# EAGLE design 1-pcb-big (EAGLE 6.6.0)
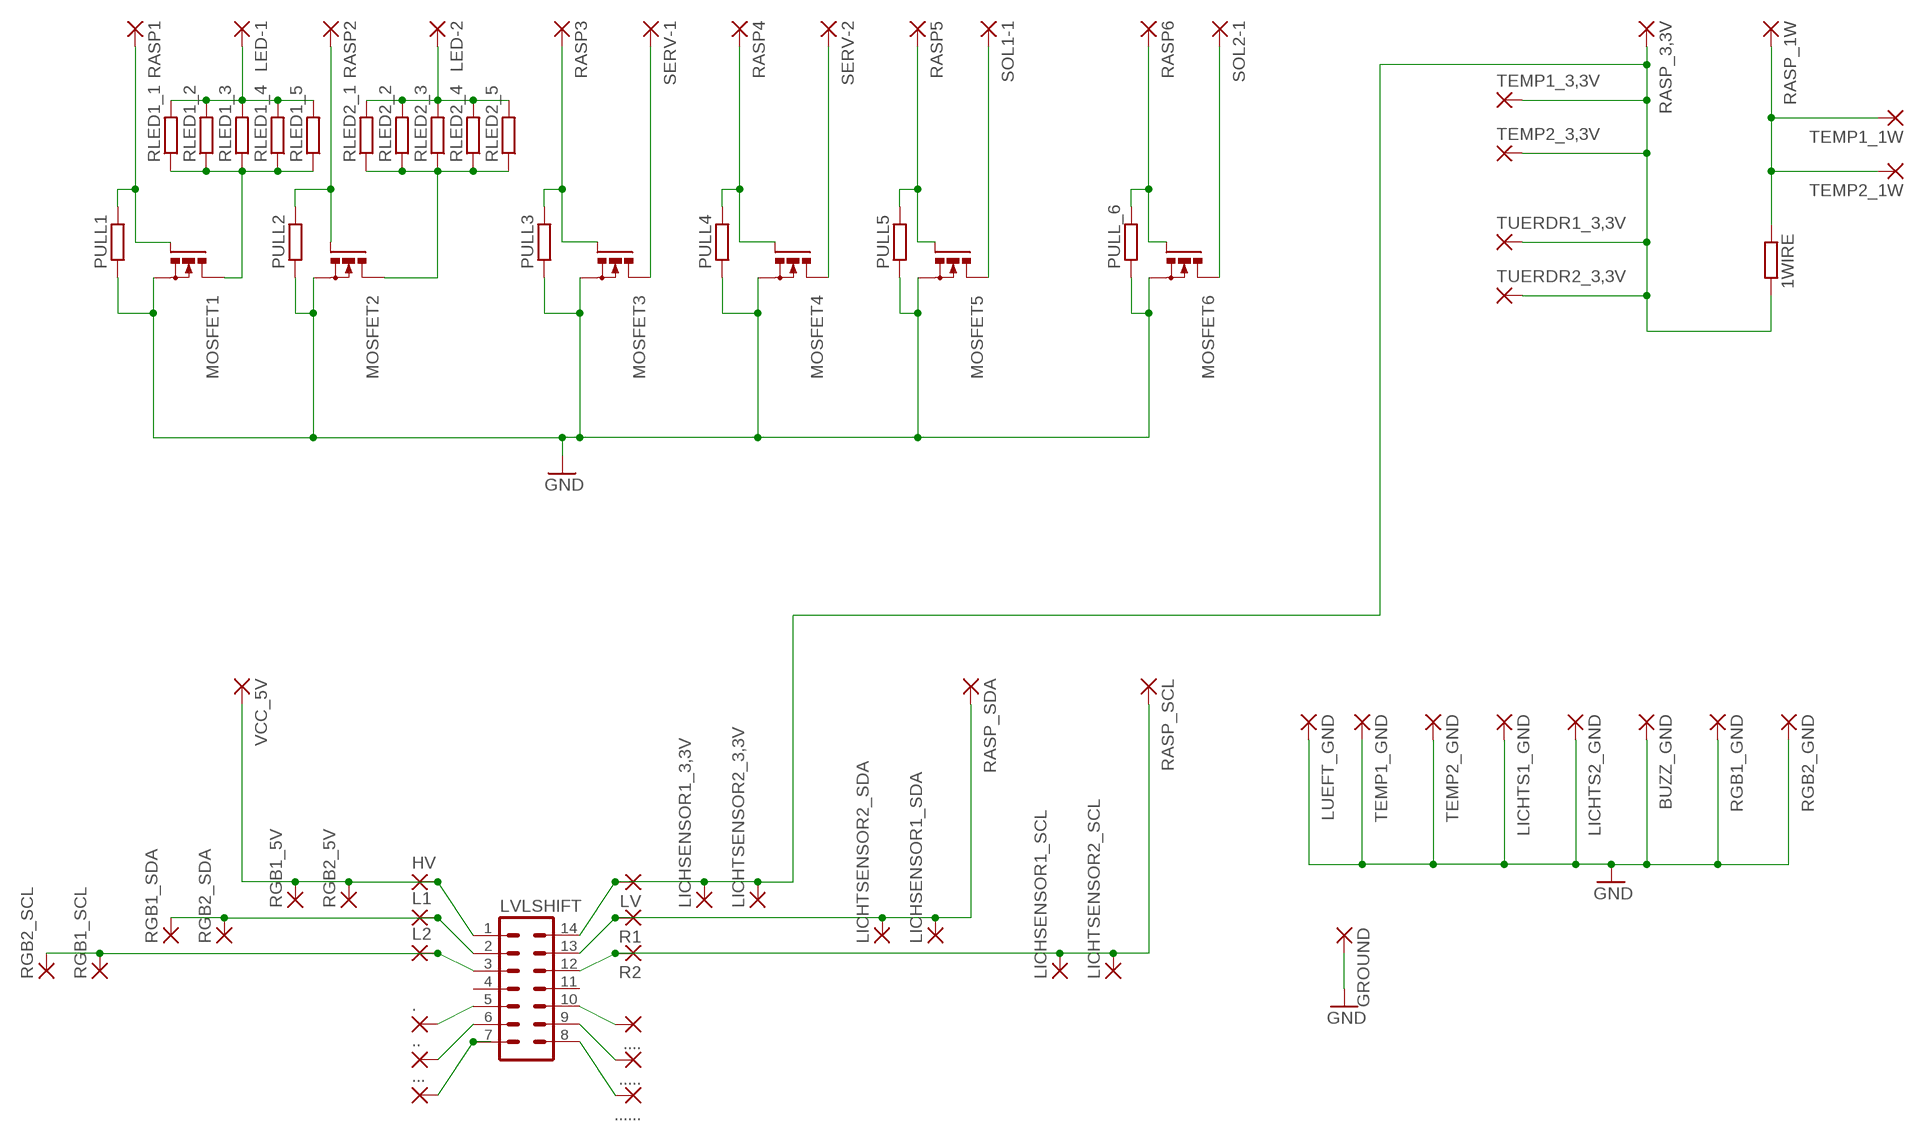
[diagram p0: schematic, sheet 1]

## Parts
1WIRE  R-EU_0207/15  [0207/15]
.  2,15/1,0  [2,15/1,0]
..  2,15/1,0  [2,15/1,0]
...  2,15/1,0  [2,15/1,0]
....  2,15/1,0  [2,15/1,0]
.....  2,15/1,0  [2,15/1,0]
......  2,15/1,0  [2,15/1,0]
BUZZ_GND  2,15/1,0  [2,15/1,0]
GROUND  2,15/1,0  [2,15/1,0]
HV  2,15/1,0  [2,15/1,0]
L1  2,15/1,0  [2,15/1,0]
L2  2,15/1,0  [2,15/1,0]
LED-1  2,15/1,0  [2,15/1,0]
LED-2  2,15/1,0  [2,15/1,0]
LICHSENSOR1_3,3V  2,15/1,0  [2,15/1,0]
LICHSENSOR1_SCL  2,15/1,0  [2,15/1,0]
LICHSENSOR1_SDA  2,15/1,0  [2,15/1,0]
LICHTS1_GND  2,15/1,0  [2,15/1,0]
LICHTS2_GND  2,15/1,0  [2,15/1,0]
LICHTSENSOR2_3,3V  2,15/1,0  [2,15/1,0]
LICHTSENSOR2_SCL  2,15/1,0  [2,15/1,0]
LICHTSENSOR2_SDA  2,15/1,0  [2,15/1,0]
LUEFT_GND  2,15/1,0  [2,15/1,0]
LV  2,15/1,0  [2,15/1,0]
LVLSHIFT  IC14P  [IC14P]
MOSFET1  BUZ11BV  [TO220BV]
MOSFET2  BUZ11BV  [TO220BV]
MOSFET3  BUZ11BV  [TO220BV]
MOSFET4  BUZ11BV  [TO220BV]
MOSFET5  BUZ11BV  [TO220BV]
MOSFET6  BUZ11BV  [TO220BV]
PULL1  R-EU_0207/10  [0207/10]
PULL2  R-EU_0207/10  [0207/10]
PULL3  R-EU_0207/10  [0207/10]
PULL4  R-EU_0207/10  [0207/10]
PULL5  R-EU_0207/10  [0207/10]
PULL_6  R-EU_0207/10  [0207/10]
R1  2,15/1,0  [2,15/1,0]
R2  2,15/1,0  [2,15/1,0]
RASP1  2,15/1,0  [2,15/1,0]
RASP2  2,15/1,0  [2,15/1,0]
RASP3  2,15/1,0  [2,15/1,0]
RASP4  2,15/1,0  [2,15/1,0]
RASP5  2,15/1,0  [2,15/1,0]
RASP6  2,15/1,0  [2,15/1,0]
RASP_1W  2,15/1,0  [2,15/1,0]
RASP_3,3V  2,15/1,0  [2,15/1,0]
RASP_SCL  2,15/1,0  [2,15/1,0]
RASP_SDA  2,15/1,0  [2,15/1,0]
RGB1_5V  2,15/1,0  [2,15/1,0]
RGB1_GND  2,15/1,0  [2,15/1,0]
RGB1_SCL  2,15/1,0  [2,15/1,0]
RGB1_SDA  2,15/1,0  [2,15/1,0]
RGB2_5V  2,15/1,0  [2,15/1,0]
RGB2_GND  2,15/1,0  [2,15/1,0]
RGB2_SCL  2,15/1,0  [2,15/1,0]
RGB2_SDA  2,15/1,0  [2,15/1,0]
RLED1_1  R-EU_0207/15  [0207/15]
RLED1_2  R-EU_0207/15  [0207/15]
RLED1_3  R-EU_0207/15  [0207/15]
RLED1_4  R-EU_0207/15  [0207/15]
RLED1_5  R-EU_0207/15  [0207/15]
RLED2_1  R-EU_0207/15  [0207/15]
RLED2_2  R-EU_0207/15  [0207/15]
RLED2_3  R-EU_0207/15  [0207/15]
RLED2_4  R-EU_0207/15  [0207/15]
RLED2_5  R-EU_0207/15  [0207/15]
SERV-1  2,15/1,0  [2,15/1,0]
SERV-2  2,15/1,0  [2,15/1,0]
SOL1-1  2,15/1,0  [2,15/1,0]
SOL2-1  2,15/1,0  [2,15/1,0]
TEMP1_1W  2,15/1,0  [2,15/1,0]
TEMP1_3,3V  2,15/1,0  [2,15/1,0]
TEMP1_GND  2,15/1,0  [2,15/1,0]
TEMP2_1W  2,15/1,0  [2,15/1,0]
TEMP2_3,3V  2,15/1,0  [2,15/1,0]
TEMP2_GND  2,15/1,0  [2,15/1,0]
TUERDR1_3,3V  2,15/1,0  [2,15/1,0]
TUERDR2_3,3V  2,15/1,0  [2,15/1,0]
VCC_5V  2,15/1,0  [2,15/1,0]

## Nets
GND: BUZZ_GND.1(P) GROUND.1(P) LICHTS1_GND.1(P) LICHTS2_GND.1(P) LUEFT_GND.1(P) MOSFET1.S MOSFET2.S MOSFET3.S MOSFET4.S MOSFET5.S MOSFET6.S PULL1.1 PULL2.1 PULL3.1 PULL4.1 PULL5.1 PULL_6.1 RGB1_GND.1(P) RGB2_GND.1(P) TEMP1_GND.1(P) TEMP2_GND.1(P)
N$1: HV.1(P) LVLSHIFT.1 RGB1_5V.1(P) RGB2_5V.1(P) VCC_5V.1(P)
N$2: MOSFET1.D RLED1_1.1 RLED1_2.1 RLED1_3.1 RLED1_4.1 RLED1_5.1
N$3: LED-2.1(P) RLED2_1.2 RLED2_2.2 RLED2_3.2 RLED2_4.2 RLED2_5.2
N$5: 1WIRE.2 LICHSENSOR1_3,3V.1(P) LICHTSENSOR2_3,3V.1(P) LV.1(P) LVLSHIFT.14 RASP_3,3V.1(P) TEMP1_3,3V.1(P) TEMP2_3,3V.1(P) TUERDR1_3,3V.1(P) TUERDR2_3,3V.1(P)
N$6: MOSFET2.G PULL2.2 RASP2.1(P)
N$7: LED-1.1(P) RLED1_1.2 RLED1_2.2 RLED1_3.2 RLED1_4.2 RLED1_5.2
N$8: MOSFET1.G PULL1.2 RASP1.1(P)
N$10: MOSFET3.D SERV-1.1(P)
N$11: MOSFET4.G PULL4.2 RASP4.1(P)
N$13: MOSFET4.D SERV-2.1(P)
N$14: MOSFET5.G PULL5.2 RASP5.1(P)
N$15: MOSFET3.G PULL3.2 RASP3.1(P)
N$16: MOSFET5.D SOL1-1.1(P)
N$17: MOSFET6.G PULL_6.2 RASP6.1(P)
N$18: ..1(P) LVLSHIFT.5
N$19: ...1(P) LVLSHIFT.6
N$21: ....1(P) LVLSHIFT.7
N$22: .......1(P) LVLSHIFT.8
N$23: ......1(P) LVLSHIFT.9
N$24: .....1(P) LVLSHIFT.10
N$25: L1.1(P) LVLSHIFT.2 RGB1_SDA.1(P) RGB2_SDA.1(P)
N$27: LICHSENSOR1_SCL.1(P) LICHTSENSOR2_SCL.1(P) LVLSHIFT.12 R2.1(P) RASP_SCL.1(P)
N$28: MOSFET6.D SOL2-1.1(P)
N$29: LICHSENSOR1_SDA.1(P) LICHTSENSOR2_SDA.1(P) LVLSHIFT.13 R1.1(P) RASP_SDA.1(P)
N$30: 1WIRE.1 RASP_1W.1(P) TEMP1_1W.1(P) TEMP2_1W.1(P)
N$33: L2.1(P) LVLSHIFT.3 RGB1_SCL.1(P) RGB2_SCL.1(P)
RLED2_3: MOSFET2.D RLED2_1.1 RLED2_2.1 RLED2_3.1 RLED2_4.1 RLED2_5.1
Unconnected: LVLSHIFT.4 LVLSHIFT.11

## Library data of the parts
1WIRE RLED1_1-RLED1_5 RLED2_1-RLED2_5 = resistor:R-EU_: RESISTOR, European symbol
. .. ... .... ..... ...... BUZZ_GND GROUND HV L1 L2 LED-1 LED-2 LICHSENSOR1_3,3V LICHSENSOR1_SCL LICHSENSOR1_SDA LICHTS1_GND LICHTS2_GND LICHTSENSOR2_3,3V LICHTSENSOR2_SCL LICHTSENSOR2_SDA LUEFT_GND LV R1 R2 RASP1-RASP6 RASP_1W RASP_3,3V RASP_SCL RASP_SDA RGB1_5V RGB1_GND RGB1_SCL RGB1_SDA RGB2_5V RGB2_GND RGB2_SCL RGB2_SDA SERV-1 SERV-2 SOL1-1 SOL2-1 TEMP1_1W TEMP1_3,3V TEMP1_GND TEMP2_1W TEMP2_3,3V TEMP2_GND TUERDR1_3,3V TUERDR2_3,3V VCC_5V = wirepad:2,15/1,0: THROUGH-HOLE PAD
LVLSHIFT = con-dil:IC14P: DIL CABLE CONNECTOR
MOSFET1-MOSFET6 = transistor-power:BUZ11: N-CHANNEL MOS FET
PULL1-PULL5 PULL_6 = rcl:R-EU_: RESISTOR, European symbol

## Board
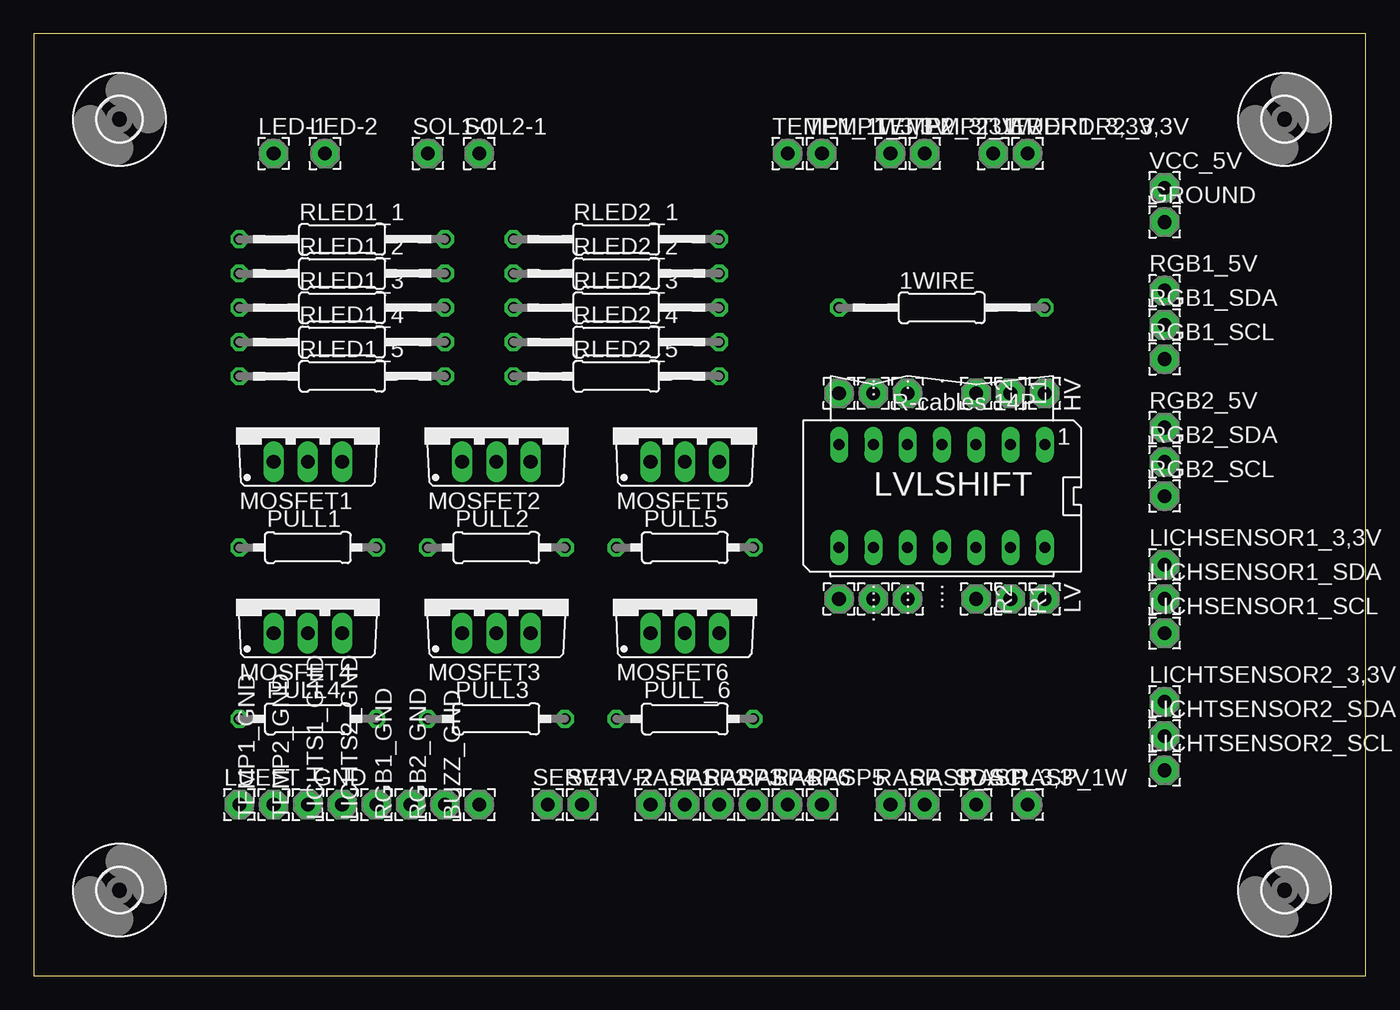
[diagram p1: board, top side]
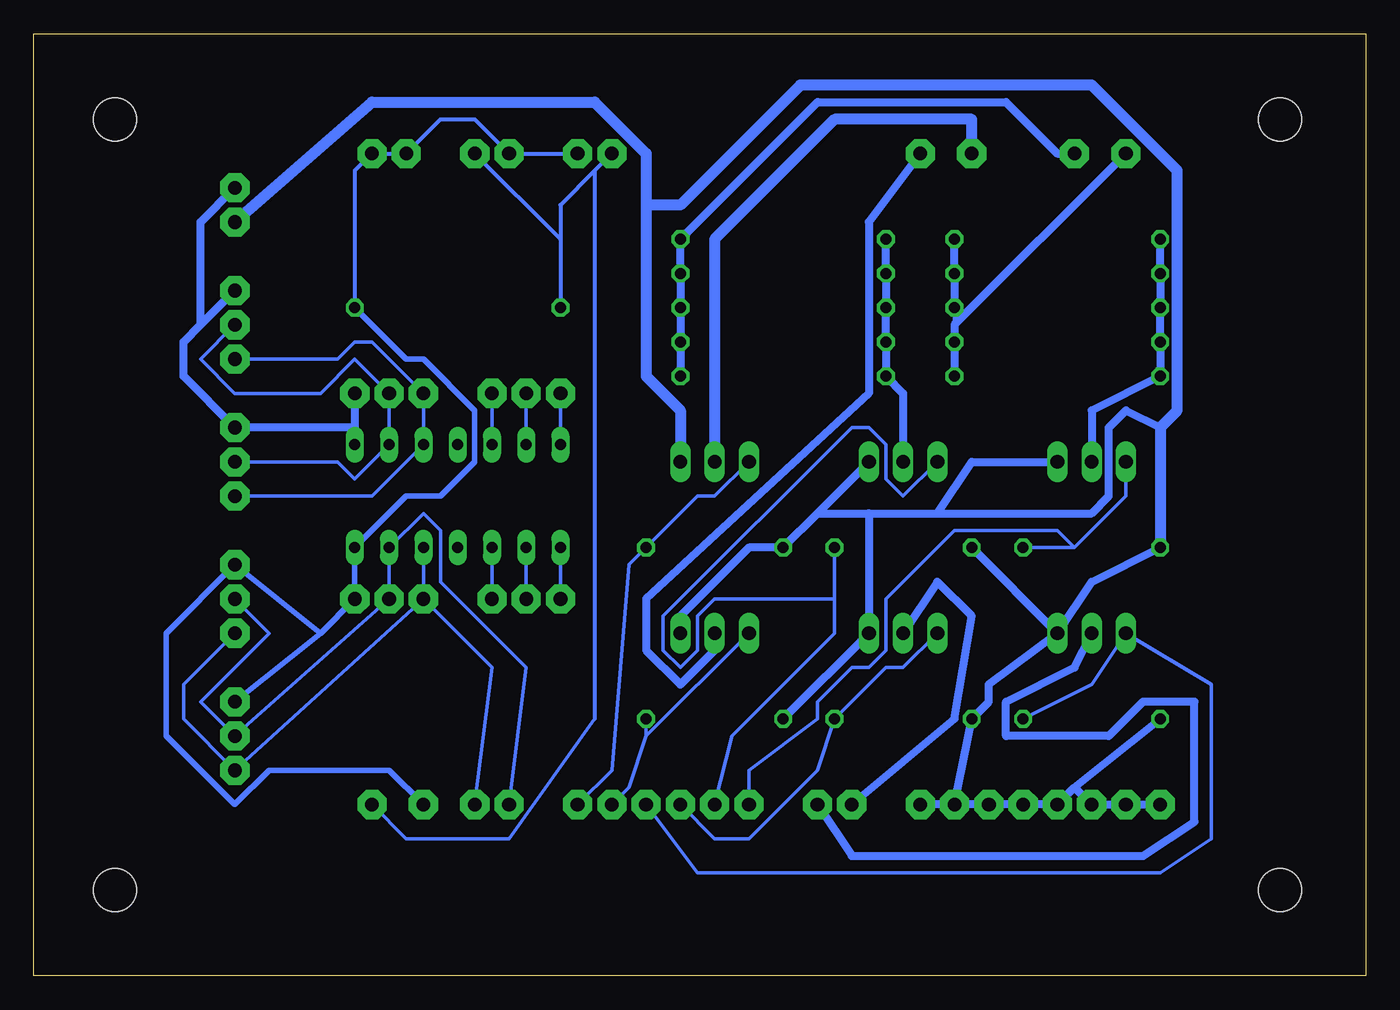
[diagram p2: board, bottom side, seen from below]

Size 98.73 x 69.84 mm. Coordinates in mm from the lower left corner, seen from the top.
Outline: 0,0 98.73,0 98.73,69.84 0,69.84 0,0
Copper layers (1*16): Top 0.035mm / dielectric 1.5mm / Bottom 0.035mm
Design rules "default": minimum track width 10mil, minimum drill 24mil, track to track 8mil, track to pad 8mil, pad to pad 8mil, via to via 8mil, smd to smd 8mil, copper to edge 40mil, drill to drill 8mil, minimum pad ring 10mil, minimum via ring 8mil, stop-mask expansion 4mil, vias tented up to drill 0mil, thermal gap 10mil

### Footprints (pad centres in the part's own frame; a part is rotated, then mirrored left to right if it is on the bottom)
0207/15 = drill 0.813 octagon: 1 -7.62,0; 2 7.62,0
2,15/1,0 = drill 1.016 pad 2.159 octagon: 1 0,0
IC14P = drill 0.813 long: 1 -7.62,-3.81; 2 -5.08,-3.81; 3 -2.54,-3.81; 4 0,-3.81; 5 2.54,-3.81; 6 5.08,-3.81; 7 7.62,-3.81; 8 7.62,3.81; 9 5.08,3.81; 10 2.54,3.81; 11 0,3.81; 12 -2.54,3.81; 13 -5.08,3.81; 14 -7.62,3.81
TO220BV = drill 1.016 long: D 0,-2.54; G -2.54,-2.54; S 2.54,-2.54
0207/10 = drill 0.813 octagon: 1 -5.08,0; 2 5.08,0
3,2 = hole 3.2: 0,0

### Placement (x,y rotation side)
1WIRE  67.31,49.53 0 top
.  64.77,43.18 270 top
..  62.23,43.18 270 top
...  59.69,43.18 270 top
....  64.77,27.94 270 top
.....  62.23,27.94 270 top
......  59.69,27.94 270 top
BUZZ_GND  33.02,12.7 90 top
GROUND  83.82,55.88 0 top
HV  74.93,43.18 270 top
L1  72.39,43.18 270 top
L2  69.85,43.18 270 top
LED-1  17.78,60.96 0 top
LED-2  21.59,60.96 0 top
LICHSENSOR1_3,3V  83.82,30.48 0 top
LICHSENSOR1_SCL  83.82,25.4 0 top
LICHSENSOR1_SDA  83.82,27.94 0 top
LICHTS1_GND  22.86,12.7 90 top
LICHTS2_GND  25.4,12.7 90 top
LICHTSENSOR2_3,3V  83.82,20.32 0 top
LICHTSENSOR2_SCL  83.82,15.24 0 top
LICHTSENSOR2_SDA  83.82,17.78 0 top
LUEFT_GND  15.24,12.7 0 top
LV  74.93,27.94 270 top
LVLSHIFT  67.31,35.56 180 top
MOSFET1  20.32,40.64 0 top
MOSFET2  34.29,40.64 0 top
MOSFET3  34.29,27.94 0 top
MOSFET4  20.32,27.94 0 top
MOSFET5  48.26,40.64 0 top
MOSFET6  48.26,27.94 0 top
PULL1  20.32,31.75 0 top
PULL2  34.29,31.75 0 top
PULL3  34.29,19.05 0 top
PULL4  20.32,19.05 0 top
PULL5  48.26,31.75 0 top
PULL_6  48.26,19.05 0 top
R1  72.39,27.94 270 top
R2  69.85,27.94 270 top
RASP1  45.72,12.7 0 top
RASP2  48.26,12.7 0 top
RASP3  50.8,12.7 0 top
RASP4  53.34,12.7 0 top
RASP5  58.42,12.7 0 top
RASP6  55.88,12.7 0 top
RASP_1W  73.66,12.7 0 top
RASP_3,3V  69.85,12.7 0 top
RASP_SCL  66.04,12.7 0 top
RASP_SDA  63.5,12.7 0 top
RGB1_5V  83.82,50.8 0 top
RGB1_GND  27.94,12.7 90 top
RGB1_SCL  83.82,45.72 0 top
RGB1_SDA  83.82,48.26 0 top
RGB2_5V  83.82,40.64 0 top
RGB2_GND  30.48,12.7 90 top
RGB2_SCL  83.82,35.56 0 top
RGB2_SDA  83.82,38.1 0 top
RLED1_1  22.86,54.61 0 top
RLED1_2  22.86,52.07 0 top
RLED1_3  22.86,49.53 0 top
RLED1_4  22.86,46.99 0 top
RLED1_5  22.86,44.45 0 top
RLED2_1  43.18,54.61 0 top
RLED2_2  43.18,52.07 0 top
RLED2_3  43.18,49.53 0 top
RLED2_4  43.18,46.99 0 top
RLED2_5  43.18,44.45 0 top
SERV-1  38.1,12.7 0 top
SERV-2  40.64,12.7 0 top
SOL1-1  29.21,60.96 0 top
SOL2-1  33.02,60.96 0 top
TEMP1_1W  55.88,60.96 0 top
TEMP1_3,3V  58.42,60.96 0 top
TEMP1_GND  17.78,12.7 90 top
TEMP2_1W  66.04,60.96 0 top
TEMP2_3,3V  63.5,60.96 0 top
TEMP2_GND  20.32,12.7 90 top
TUERDR1_3,3V  71.12,60.96 0 top
TUERDR2_3,3V  73.66,60.96 0 top
U$1  [3,2]  92.71,63.5 0 top
U$2  [3,2]  6.35,63.5 0 top
U$3  [3,2]  6.35,6.35 0 top
U$4  [3,2]  92.71,6.35 0 top
VCC_5V  83.82,58.42 0 top

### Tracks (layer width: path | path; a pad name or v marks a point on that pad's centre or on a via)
GND
  Bottom 0.61: PULL1.1 20.32,29.21 MOSFET4.S | MOSFET4.S PULL2.1 | RGB2_GND.1 PULL3.1 27.94,20.32 27.94,21.59 MOSFET4.S | RGB2_GND.1 BUZZ_GND.1 | 21.59,13.97 LICHTS1_GND.1 LICHTS2_GND.1 RGB1_GND.1 RGB2_GND.1 | 21.59,13.97 PULL4.1 | 21.59,13.97 TEMP2_GND.1 TEMP1_GND.1 LUEFT_GND.1 | PULL_6.1 MOSFET3.S 36.83,34.29 | MOSFET2.S 40.64,34.29 | 40.64,34.29 PULL5.1 45.72,31.75 50.8,26.67 MOSFET6.S | MOSFET1.S 29.21,38.1 31.75,34.29 | 40.64,34.29 36.83,34.29 | 36.83,34.29 31.75,34.29 | 15.24,40.64 17.78,41.91 19.05,40.64 19.05,35.56 20.32,34.29 31.75,34.29
  Bottom 0.813: MOSFET5.S 50.8,41.91 53.34,44.45 53.34,57.15 | 53.34,57.15 53.34,60.96 57.15,64.77 73.66,64.77 GROUND.1 | PULL1.1 15.24,40.64 13.97,41.91 13.97,59.69 20.32,66.04 41.91,66.04 50.8,57.15 53.34,57.15
N$1
  Bottom 0.254: 74.93,40.64 LVLSHIFT.1
  Bottom 0.61: HV.1 74.93,40.64 RGB2_5V.1 87.63,44.45 87.63,46.99 86.36,48.26 | 86.36,48.26 RGB1_5V.1 | VCC_5V.1 86.36,55.88 86.36,48.26
N$2
  Bottom 0.61: RLED1_1.1 RLED1_2.1 RLED1_3.1 RLED1_4.1 RLED1_5.1 20.32,41.91 MOSFET1.D
N$3
  Bottom 0.61: RLED2_5.2 RLED2_4.2 RLED2_3.2 RLED2_2.2 RLED2_1.2 40.64,64.77 26.67,64.77 22.86,60.96 LED-2.1
N$5
  Bottom 0.305: TEMP1_3,3V.1 TEMP2_3,3V.1 66.04,63.5 68.58,63.5 TUERDR1_3,3V.1 TUERDR2_3,3V.1 74.93,59.69 1WIRE.2
  Bottom 0.406: 77.47,25.4 LV.1 LVLSHIFT.14 71.12,35.56 68.58,35.56 66.04,38.1 66.04,41.91 69.85,45.72 71.12,45.72 1WIRE.2 | 77.47,25.4 LICHTSENSOR2_3,3V.1 | RASP_3,3V.1 72.39,15.24 77.47,15.24 81.28,15.24 83.82,12.7 88.9,17.78 88.9,25.4 LICHSENSOR1_3,3V.1 77.47,25.4
N$6
  Bottom 0.254: 39.37,27.94 39.37,25.4 46.99,17.78 RASP2.1 | 39.37,27.94 PULL2.2 | MOSFET2.G 34.29,35.56 35.56,36.83 35.56,39.37 36.83,40.64 38.1,40.64 52.07,26.67 52.07,24.13 50.8,22.86 49.53,24.13 49.53,26.67 48.26,27.94 39.37,27.94
N$7
  Bottom 0.254: RLED1_3.2 30.48,48.26
  Bottom 0.61: RLED1_5.2 RLED1_4.2 30.48,48.26 LED-1.1 | RLED1_3.2 RLED1_2.2 RLED1_1.2
N$8
  Bottom 0.254: 21.59,31.75 PULL1.2 | 21.59,31.75 17.78,35.56 MOSFET1.G | RASP1.1 45.72,15.24 40.64,19.05 40.64,20.32 38.1,22.86 36.83,22.86 35.56,24.13 35.56,27.94 30.48,33.02 22.86,33.02 21.59,31.75
N$10
  Bottom 0.61: MOSFET3.D 31.75,29.21 29.21,26.67 30.48,19.05 SERV-1.1
N$11
  Bottom 0.254: PULL4.2 20.32,21.59 MOSFET4.G 11.43,21.59 11.43,10.16 15.24,7.62 49.53,7.62 RASP4.1
N$13
  Bottom 0.61: MOSFET4.D 21.59,22.86 26.67,20.32 26.67,17.78 19.05,17.78 16.51,20.32 12.7,20.32 12.7,11.43 16.51,8.89 38.1,8.89 SERV-2.1
N$14
  Bottom 0.254: MOSFET5.G 48.26,35.56 49.53,35.56 PULL5.2 54.61,30.48 55.88,15.24 RASP5.1
N$15
  Bottom 0.254: MOSFET3.G 34.29,22.86 35.56,22.86 PULL3.2 40.64,15.24 45.72,10.16 48.26,10.16 RASP3.1
N$16
  Bottom 0.813: MOSFET5.D 48.26,54.61 39.37,63.5 29.21,63.5 SOL1-1.1
N$17
  Bottom 0.254: 53.34,17.78 54.61,13.97 RASP6.1 | 53.34,17.78 PULL_6.2 | 53.34,17.78 MOSFET6.G
N$18
  Bottom 0.254: ..1 LVLSHIFT.5
N$19
  Bottom 0.254: ...1 LVLSHIFT.6
N$21
  Bottom 0.254: ....1 LVLSHIFT.7
N$22
  Bottom 0.254: .......1 LVLSHIFT.8
N$23
  Bottom 0.254: ......1 LVLSHIFT.9
N$24
  Bottom 0.254: .....1 LVLSHIFT.10
N$25
  Bottom 0.254: RGB2_SDA.1 76.2,38.1 74.93,36.83 LVLSHIFT.2 L1.1 74.93,45.72 77.47,43.18 83.82,43.18 86.36,45.72 RGB1_SDA.1
N$27
  Bottom 0.254: R2.1 LVLSHIFT.12 | RASP_SCL.1 64.77,22.86 R2.1 | R2.1 LICHTSENSOR2_SCL.1 87.63,19.05 87.63,21.59 LICHSENSOR1_SCL.1
N$28
  Bottom 0.61: MOSFET6.D 48.26,24.13 50.8,21.59 53.34,24.13 53.34,27.94 36.83,43.18 36.83,55.88 SOL2-1.1
N$29
  Bottom 0.254: RASP_SDA.1 62.23,22.86 68.58,29.21 68.58,33.02 69.85,34.29 LVLSHIFT.13 R1.1 LICHTSENSOR2_SDA.1 86.36,20.32 81.28,25.4 LICHSENSOR1_SDA.1
N$30
  Bottom 0.254: RASP_1W.1 71.12,10.16 63.5,10.16 57.15,19.05
  Bottom 0.305: 59.69,54.61 59.69,57.15 57.15,59.69 | 59.69,54.61 1WIRE.1 | TEMP1_1W.1 57.15,59.69 | 59.69,54.61 TEMP2_1W.1 | 57.15,59.69 57.15,19.05
N$33
  Bottom 0.254: RGB2_SCL.1 73.66,35.56 LVLSHIFT.3 L2.1 73.66,46.99 74.93,46.99 76.2,45.72 RGB1_SCL.1
RLED2_3
  Bottom 0.61: RLED2_1.1 RLED2_2.1 RLED2_3.1 RLED2_4.1 RLED2_5.1 34.29,43.18 MOSFET2.D

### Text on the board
Beschriftungen: LED Gruppen | Solenoids | Temp1 | Temp2 | Tuerdr3v3 | 1 | 2 | I | A | 1W | 3v3 | 3v3 | 1W | I | A | 5V | GND | 5V | RGB-LEDA | SDA | Hv | 1 | 2 | 2 | 1 | Hv | SCL | 5V | RGB-LEDI | SDA | SCL | 3v3 | LichtSA | SDA | Lv | 1 | 2 | 2 | 1 | Lv | SCL | 3v3 | LichtSI | SDA | Ground | Servos | Raspberry | SCL | LU | T1 | T2 | LI | LA | RI | RA | B | I | A | G1 | G2 | SI | SA | OI | OA | SDA | SLC | 3v3 | 1W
